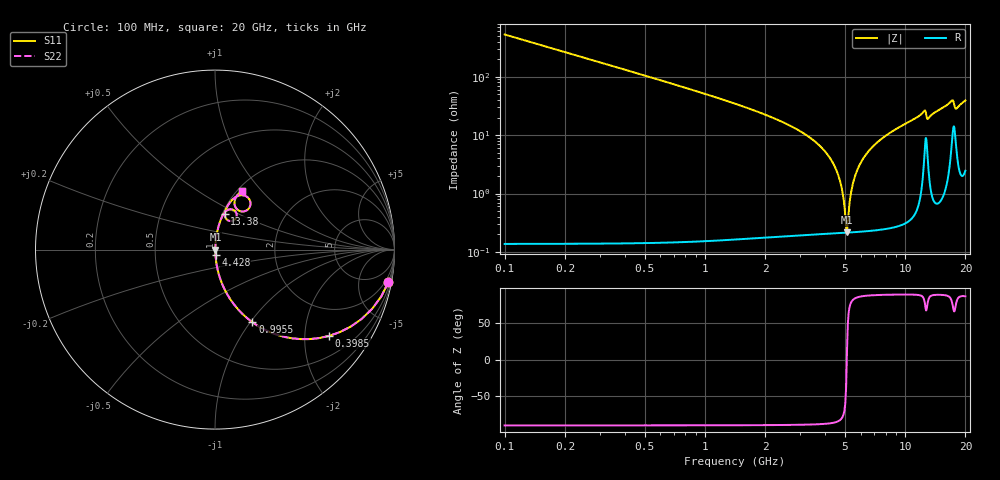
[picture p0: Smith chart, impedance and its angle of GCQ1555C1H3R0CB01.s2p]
!Murata Part Number: GCQ1555C1H3R0CB01
!These Parameters are Measured in Series Mode Connection
!Data Generated on Jan 08, 2026
!  o--ll--o
!Port1  Port2
!  o------o
!Operation Temp=25[degC], DC Bias Voltage=0[V]
!Freq. Start=100[MHz] Stop=20[GHz] 401[Steps]
# Hz S RI R 50
!Freq.(Hz) S11(Real) S11(Imag) S21(Real) S21(Imag) S12(Real) S12(Imag) S22(Real) S22(Imag)
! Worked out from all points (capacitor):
!   401 points, 100 MHz to 20 GHz, reference 50 ohm
!   read as one part in series: C = 3 pF near 199.5 MHz
!   lowest |Z| = 217 mohm at 5.125 GHz (marker M1)
!   series resonance near 5.116 GHz, so ESL is about 320 pH
!   S11 on the Smith chart (normalised r, x): 100 MHz: 1, -11; 398.5 MHz: 1.00, -2.65; 995.5 MHz: 1.00, -1.03; 4.428 GHz: 1.00, -0.06; 13.38 GHz: 1.02, +0.43; 20 GHz: 1.05, +0.78
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1e8  0.9656 -0.1821  0.0344 0.1821  0.0344 0.1821  0.9656 -0.1821
3.985e8  0.6363 -0.4805  0.3637 0.4805  0.3637 0.4805  0.6363 -0.4805
6.97e8  0.3584 -0.4785  0.6416 0.4785  0.6416 0.4785  0.3584 -0.4785
9.955e8  0.2088 -0.405  0.7912 0.405  0.7912 0.405  0.2088 -0.405
1.7915e9  0.0646 -0.2425  0.9354 0.2425  0.9354 0.2425  0.0646 -0.2425
3.43325e9  0.00911 -0.0841  0.9909 0.0841  0.9909 0.0841  0.00911 -0.0841
4.42825e9  0.00297 -0.03  0.997 0.03  0.997 0.03  0.00297 -0.03
4.7765e9  0.0023 -0.0142  0.9977 0.0142  0.9977 0.0142  0.0023 -0.0142
5.02525e9  0.00214 -0.00369  0.9979 0.00369  0.9979 0.00369  0.00214 -0.00369
5.12475e9  0.00213 0.000376  0.9979 -0.000376  0.9979 -0.000376  0.00213 0.000376
5.42325e9  0.00231 0.0121  0.9977 -0.0121  0.9977 -0.0121  0.00231 0.0121
5.672e9  0.00264 0.0215  0.9974 -0.0215  0.9974 -0.0215  0.00264 0.0215
6.11975e9  0.00363 0.0375  0.9964 -0.0375  0.9964 -0.0375  0.00363 0.0375
6.7665e9  0.00579 0.059  0.9942 -0.059  0.9942 -0.059  0.00579 0.059
1.005e10  0.027 0.1525  0.973 -0.1525  0.973 -0.1525  0.027 0.1525
1.2438e10  0.0908 0.2246  0.9092 -0.2246  0.9092 -0.2246  0.0908 0.2246
1.29355e10  0.0717 0.1633  0.9283 -0.1633  0.9283 -0.1633  0.0717 0.1633
1.338325e10  0.0543 0.1996  0.9457 -0.1996  0.9457 -0.1996  0.0543 0.1996
1.67165e10  0.1355 0.3016  0.8645 -0.3016  0.8645 -0.3016  0.1355 0.3016
1.7413e10  0.1978 0.2525  0.8022 -0.2525  0.8022 -0.2525  0.1978 0.2525
1.79105e10  0.1256 0.2222  0.8744 -0.2222  0.8744 -0.2222  0.1256 0.2222
2e10  0.1487 0.3258  0.8513 -0.3258  0.8513 -0.3258  0.1487 0.3258
